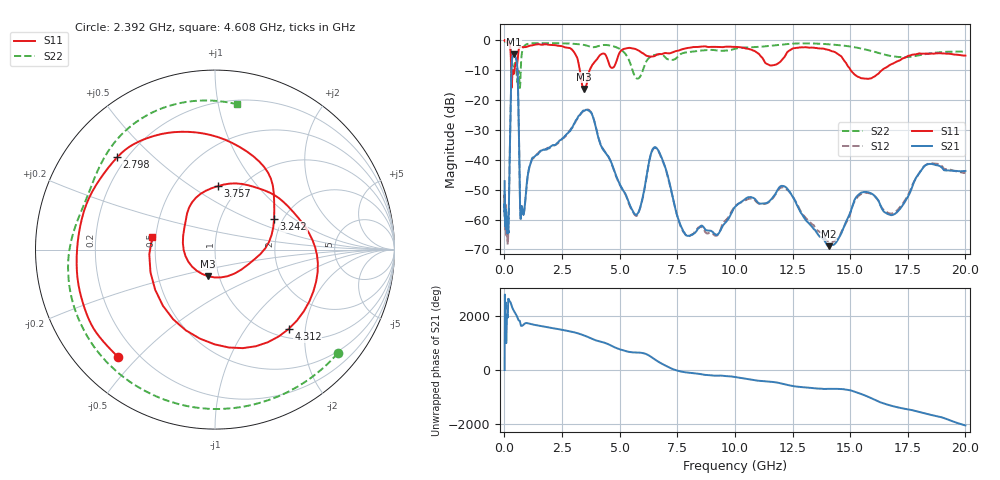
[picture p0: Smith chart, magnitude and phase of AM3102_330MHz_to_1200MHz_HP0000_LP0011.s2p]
! Date/Time: Tue, Sep 11, 2018 5:08 PM
! Network Analyzer: Agilent Technologies E8362B Rev: A.07.50.63
! Sweep from 0.010 to 20.000 GHz, 1601 Points, Sweep Type: LOG
! Power Supply: 4.950 V, 0.001 A
# Hz S DB R 50
!freq MagS11 AngS11 MagS21 AngS21 MagS12 AngS12 MagS22 AngS22
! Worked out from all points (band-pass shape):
!   1601 points, 10 MHz to 20 GHz, reference 50 ohm
!   highest |S21| = -4.67 dB at 406.7 MHz (marker M1); lowest = -68.9 dB at 14.07 GHz (marker M2)
!   |S21| within 3 dB of the highest: 317.6 MHz to 547.4 MHz (229.9 MHz wide, 53.1 % of centre)
!   lowest |S11| = -16.3 dB at 3.449 GHz (marker M3), VSWR 1.36, Z = 44.4 - j13.5 ohm
!   |S11| at or under -10 dB: 369.2 MHz to 434.7 MHz (65.47 MHz wide, 16.3 % of centre); 3.28 GHz to 3.697 GHz (416.6 MHz wide, 11.9 % of centre); 15.03 GHz to 16.38 GHz (1.351 GHz wide, 8.6 % of centre)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
!   |S22| runs from -15.9 to -0.2 dB; largest |S21 - S12| = 0.0091
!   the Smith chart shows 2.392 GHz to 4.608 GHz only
!   S11 on the Smith chart (normalised r, x): 2.392 GHz: 0.13, -0.44; 2.798 GHz: 0.17, +0.39; 3.242 GHz: 1.80, +0.71; 3.757 GHz: 0.80, +0.65; 4.312 GHz: 1.17, -1.63; 4.608 GHz: 0.48, +0.08
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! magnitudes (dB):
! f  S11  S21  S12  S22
! 10 MHz  0.0  -47.1  -51.8  -0.2
! 35.55 MHz  0.0  -60.5  -59.5  -0.4
! 126.4 MHz  -0.4  -61.8  -61.3  -0.9
! 175.4 MHz  -0.9  -63.8  -61.7  -1.2
! 406.7 MHz  -11.2  -4.7  -4.7  -9.1
! 447.2 MHz  -9.3  -5.0  -5.1  -7.7
! 572.5 MHz  -6.8  -11.0  -11.1  -13.4
! 702.3 MHz  -2.2  -59.4  -59.9  -11.7
! 1.59 GHz  -1.4  -36.9  -37.0  -0.9
! 2.392 GHz  -1.9  -33.5  -33.9  -1.0
! 2.798 GHz  -2.5  -30.6  -30.6  -1.0
! 3.242 GHz  -8.6  -25.2  -25.3  -1.3
! 3.449 GHz  -16.3  -23.5  -23.5  -1.5
! 3.757 GHz  -9.0  -24.1  -24.0  -2.2
! 4.312 GHz  -4.4  -36.8  -36.7  -1.5
! 4.608 GHz  -9.0  -40.3  -40.4  -1.7
! 5.652 GHz  -2.8  -58.2  -58.4  -11.9
! 6.58 GHz  -4.9  -35.9  -36.1  -4.8
! 7.92 GHz  -2.6  -65.4  -65.3  -4.0
! 12.09 GHz  -6.1  -48.7  -49.2  -1.4
! 14.07 GHz  -3.2  -68.9  -67.3  -1.3
! 20 GHz  -5.1  -43.7  -44.4  -3.7
